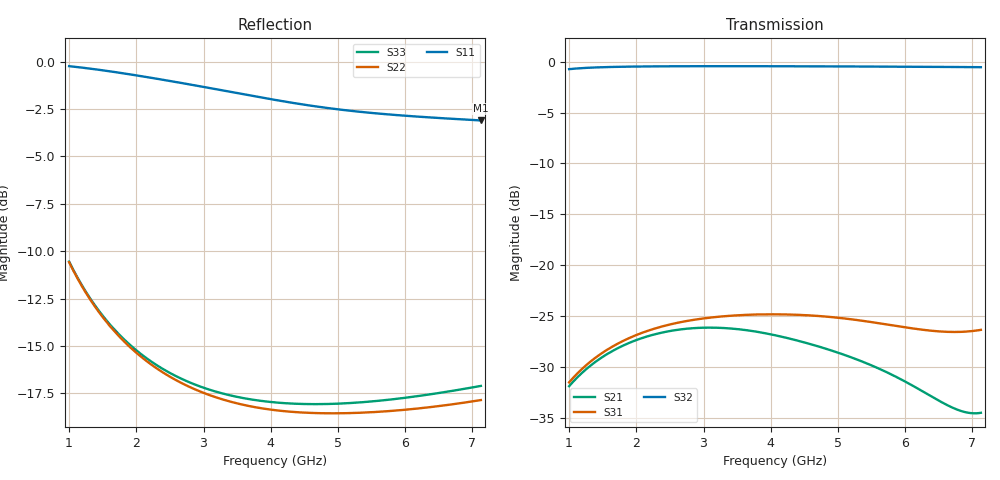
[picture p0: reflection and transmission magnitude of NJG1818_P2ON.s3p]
! Created Mon Jul  5 12:49:41 2021
# hz S ma R 50
! 3 Port Network Data from SP1.SP block
! freq  magS11  angS11  magS12  angS12  magS13  angS13
!  magS21  angS21
!  magS22  angS22  magS23  angS23
!  magS31  angS31  magS32  angS32
!  magS33  angS33
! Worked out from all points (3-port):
!   1226 points, 1 GHz to 7.125 GHz, reference 50 ohm
!   strongest paths, dB at 1 GHz, 2.53 GHz, 4.065 GHz, 5.595 GHz, 7.125 GHz:
!     S32: -0.7, -0.5, -0.5, -0.5, -0.5
!     S31: -31.5, -25.8, -24.8, -25.7, -26.4
!     S21: -31.9, -26.4, -26.9, -30.1, -34.5
!   lowest |S11| = -3.1 dB at 7.125 GHz (marker M1), VSWR 5.66, Z = 8.85 + j1.94 ohm
!   |S11| at or under -10 dB: nowhere
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1e9  0.9726 -36.2  0.02546 66.2  0.02658 70.8
     0.02546 66.2  0.2957 -73.2  0.9182 10.8
     0.02658 70.8  0.9182 10.8  0.2968 -73.1
1.665e9  0.9394 -58.8  0.03822 52.1  0.0402 59.7
         0.03822 52.1  0.1952 -80.2  0.9419 0.6
         0.0402 59.7  0.9419 0.6  0.1972 -79.9
2.34e9  0.8989 -80.0  0.04634 39.1  0.04957 50.3
        0.04634 39.1  0.1536 -84.5  0.948 -6.1
        0.04957 50.3  0.948 -6.1  0.1567 -83.9
2.76e9  0.8726 -92.3  0.0488 31.7  0.05329 45.5
        0.0488 31.7  0.1395 -87.0  0.9493 -9.6
        0.05329 45.5  0.9493 -9.6  0.1433 -86.1
3.23e9  0.8429 -105.1  0.04927 24.5  0.05587 41.2
        0.04927 24.5  0.1294 -89.8  0.9498 -13.2
        0.05587 41.2  0.9498 -13.2  0.134 -88.6
4.065e9  0.7924 -125.7  0.04528 15.0  0.05738 36.0
         0.04528 15.0  0.1204 -95.2  0.9491 -19.1
         0.05738 36.0  0.9491 -19.1  0.1262 -93.0
4.73e9  0.7591 -140.1  0.03971 11.6  0.05625 33.9
        0.03971 11.6  0.1182 -100.0  0.9478 -23.5
        0.05625 33.9  0.9478 -23.5  0.1249 -96.8
5.485e9  0.7325 -154.9  0.03235 12.3  0.05263 34.5
         0.03235 12.3  0.1189 -106.0  0.9457 -28.4
         0.05263 34.5  0.9457 -28.4  0.1269 -101.3
6.72e9  0.7061 -177.4  0.01986 36.7  0.047 48.9
        0.01986 36.7  0.1249 -116.8  0.941 -36.4
        0.047 48.9  0.941 -36.4  0.1355 -109.5
7.125e9  0.6995 175.4  0.01884 58.5  0.04814 57.5
         0.01884 58.5  0.128 -120.5  0.9389 -39.0
         0.04814 57.5  0.9389 -39.0  0.1395 -112.5
